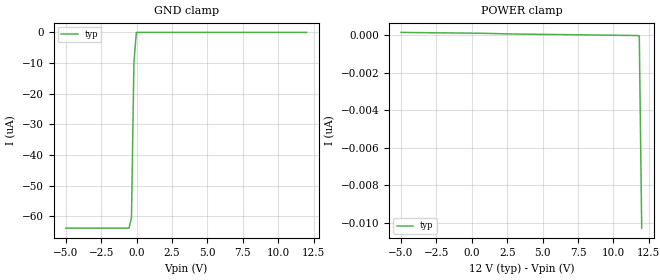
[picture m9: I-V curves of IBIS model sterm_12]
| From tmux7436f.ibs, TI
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| sterm_12
[Model]   sterm_12
Model_type   Terminator
|   typ   min   max
C_comp   4.014581e-12   NA   NA
[Voltage Range]   12   NA   NA
[Temperature Range]   27   NA   NA
[Power Clamp Reference]   12   NA   NA
[GND Clamp Reference]   0   NA   NA
[GND Clamp]
|   Voltage   I(typ)   I(min)   I(max)
-5V       -63.89uA   NA         NA
-535.4mV  -63.88uA   NA         NA
-363.6mV  -60.5uA    NA         NA
-191.9mV  -9.798uA   NA         NA
-20.2mV   -22.4nA    NA         NA
12V       103.5pA    NA         NA
[POWER Clamp]
|   Voltage   I(typ)   I(min)   I(max)
-5V       144.8pA    NA         NA
494.9mV   99.54pA    NA         NA
11.83V    -38.63pA   NA         NA
12V       -10.29nA   NA         NA
